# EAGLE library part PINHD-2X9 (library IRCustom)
PIN HEADER With larger annulars
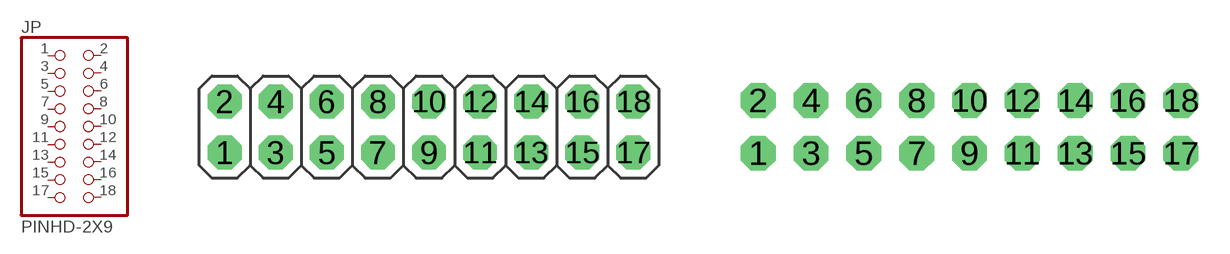
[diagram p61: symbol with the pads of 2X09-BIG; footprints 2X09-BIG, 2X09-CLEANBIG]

Designator prefix JP

## PINHD-2X9-BIG  [2X09-BIG]
1  1  pas
2  2  pas
3  3  pas
4  4  pas
5  5  pas
6  6  pas
7  7  pas
8  8  pas
9  9  pas
10  10  pas
11  11  pas
12  12  pas
13  13  pas
14  14  pas
15  15  pas
16  16  pas
17  17  pas
18  18  pas

## PINHD-2X9-CBIG  [2X09-CLEANBIG]
Pads as for 2X09-BIG

## Footprint 2X09-BIG (pad centres in mm)
PIN HEADER
drill 1.016 pad 1.676 octagon: 1 -10.16,-1.27; 2 -10.16,1.27; 3 -7.62,-1.27; 4 -7.62,1.27; 5 -5.08,-1.27; 6 -5.08,1.27; 7 -2.54,-1.27; 8 -2.54,1.27; 9 0,-1.27; 10 0,1.27; 11 2.54,-1.27; 12 2.54,1.27; 13 5.08,-1.27; 14 5.08,1.27; 15 7.62,-1.27; 16 7.62,1.27; 17 10.16,-1.27; 18 10.16,1.27

## Footprint 2X09-CLEANBIG (pad centres in mm)
drill 1.016 pad 1.676 octagon: 1 -10.16,-1.27; 2 -10.16,1.27; 3 -7.62,-1.27; 4 -7.62,1.27; 5 -5.08,-1.27; 6 -5.08,1.27; 7 -2.54,-1.27; 8 -2.54,1.27; 9 0,-1.27; 10 0,1.27; 11 2.54,-1.27; 12 2.54,1.27; 13 5.08,-1.27; 14 5.08,1.27; 15 7.62,-1.27; 16 7.62,1.27; 17 10.16,-1.27; 18 10.16,1.27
